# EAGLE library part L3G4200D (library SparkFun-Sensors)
ST Microelectronics L3G4200D 3-Axis Digital Output Gyroscope The L3G4200D is a low-power three-axis angular rate sensor, has a full scale of ±250/±500/±2000 dps and is capable of measuring rates with a user-selectable bandwidth. It includes a sensing element and an IC interface capable of providing the measured angular rate to the external world through a digital interface (I2C/SPI). Datasheet SparkFun Products SparkFun Tri-Axis Gyro Breakout - L3G4200D (SEN-10612)
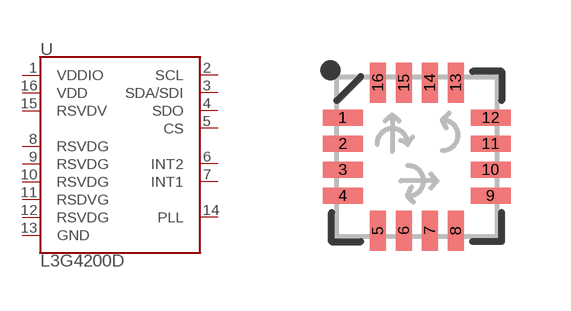
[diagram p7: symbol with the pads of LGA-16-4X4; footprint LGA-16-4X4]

Designator prefix U

## L3G4200D (PROD_ID: IC-10395)  [LGA-16-4X4]
1  VDDIO
2  SCL
3  SDA/SDI
4  SDO
5  CS
6  INT2
7  INT1
8  RSVDG
9  RSVDG
10  RSVDG
11  RSDVG
12  RSVDG
13  GND
14  PLL
15  RSVDV
16  VDD

## Footprint LGA-16-4X4 (pad centres in mm)
16-pin LGA Package Datasheet Specifications: Pin Count: 16 Area: 4.0 x 4.0 x 1.1 mm Pitch: 0.65 mm Devices Using: L3G4200D
smd 1 x 0.4: 1 -1.85,0.975; 2 -1.85,0.325; 3 -1.85,-0.325; 4 -1.85,-0.975; 9 1.85,-0.975; 10 1.85,-0.325; 11 1.85,0.325; 12 1.85,0.975
smd 0.4 x 1: 5 -0.975,-1.85; 6 -0.325,-1.85; 7 0.325,-1.85; 8 0.975,-1.85; 13 0.975,1.85; 14 0.325,1.85; 15 -0.325,1.85; 16 -0.975,1.85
